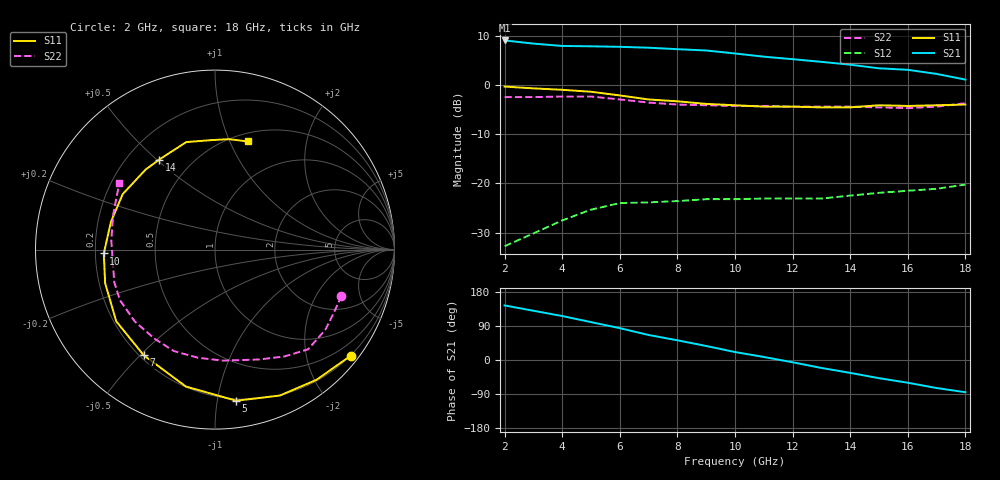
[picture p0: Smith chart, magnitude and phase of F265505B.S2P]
!ATF-26550
!S-PARAMETERS at Vds=5V  Id=30mA.  LAST UPDATED 07-22-92
# ghz s ma r 50
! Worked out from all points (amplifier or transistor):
!   17 points, 2 GHz to 18 GHz, reference 50 ohm
!   highest |S21| = 9.0 dB at 2 GHz (marker M1)
!   |S21| within 3 dB of that: start of sweep to 10.55 GHz
!   unconditionally stable (mu >= 1): 8.689 GHz to end of sweep
!   at 4 GHz: K = 0.29, MSG = 17.7 dB, |S12| = -27.5 dB
!   at 10 GHz: K = 1.18, MAG = 12.3 dB, |S12| = -23.2 dB
!   at 18 GHz: K = 1.25, MAG = 7.6 dB, |S12| = -20.3 dB
!   S11 on the Smith chart (normalised r, x): 2 GHz: 0.19, -2.89; 5 GHz: 0.19, -1.13; 7 GHz: 0.22, -0.51; 10 GHz: 0.23, -0.02; 14 GHz: 0.33, +0.51; 18 GHz: 0.59, +1.17
2  0.96 -38.0  2.82 144.0  0.023 69.0  0.75 -20.0
3  0.92 -52.0  2.62 130.0  0.031 70.0  0.75 -28.0
4  0.89 -66.0  2.48 116.0  0.042 68.0  0.76 -36.0
5  0.85 -82.0  2.46 100.0  0.054 65.0  0.76 -47.0
6  0.78 -102.0  2.43 84.0  0.063 46.0  0.71 -57.0
7  0.71 -124.0  2.38 66.0  0.064 30.0  0.66 -68.0
8  0.68 -144.0  2.3 52.0  0.066 25.0  0.63 -78.0
9  0.64 -163.0  2.23 37.0  0.069 19.0  0.62 -86.0
10  0.62 -178.0  2.08 21.0  0.069 12.0  0.61 -99.0
11  0.6 165.0  1.93 8.0  0.07 5.0  0.61 -112.0
12  0.6 149.0  1.82 -6.0  0.07 -3.0  0.6 -124.0
13  0.59 131.0  1.71 -21.0  0.07 -8.0  0.6 -138.0
14  0.59 122.0  1.6 -34.0  0.075 -15.0  0.6 -152.0
15  0.62 105.0  1.47 -48.0  0.08 -20.0  0.59 -162.0
16  0.61 93.0  1.42 -60.0  0.084 -25.0  0.58 175.0
17  0.62 83.0  1.29 -74.0  0.088 -31.0  0.6 161.0
18  0.63 73.0  1.13 -85.0  0.097 -40.0  0.65 145.0
